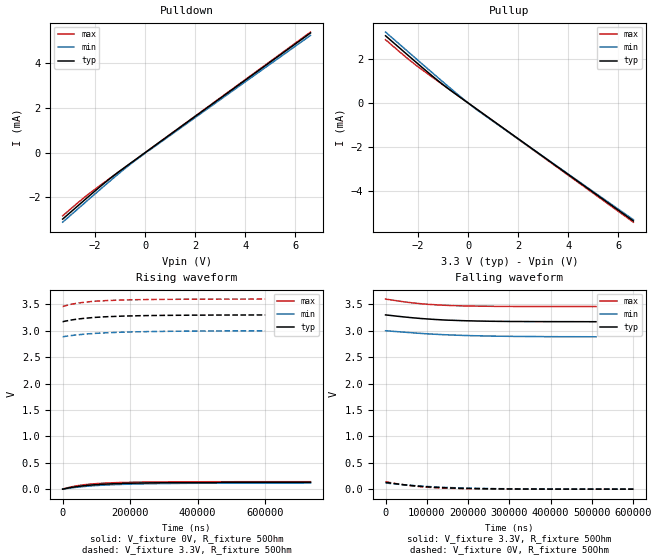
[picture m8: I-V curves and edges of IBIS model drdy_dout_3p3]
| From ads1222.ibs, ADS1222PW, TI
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|   drdy_dout_3p3 Model
[Model]   drdy_dout_3p3
Model_type   Output
Polarity   Non-Inverting
Vmeas = 1.65
Vref = 1.65
Cref = 2pF
Rref = 50
|   typ   min   max
|   (nom PVT)   (fast PVT)   (slow PVT)
|C_comp from frequency sweep method (F= 2.5MHz)
|Average
|C_comp   7.50e-15   6.37e-15   9.00e-15
|ON state : BUFFER OUTPUT TURNED HIGH
C_comp   5.929e-15   5.016e-15   7.087e-15
|OFF state: BUFFER IN HIGH IMPEDANCE
|C_comp   9.065e-15   7.724e-15   1.091e-14
|C_comp from LC tank measurement(L=1nH)
|Average
|Resonant Frequency(Hz)   1.000e+12   1.000e+12   1.000e+12
|C_comp   2.536e-17   2.536e-17   2.536e-17
|ON state : BUFFER OUTPUT TURNED HIGH
|Resonant Frequency(Hz)   1.000e+12   1.000e+12   1.000e+12
|C_comp   2.536e-17   2.536e-17   2.536e-17
|OFF state: BUFFER IN HIGH IMPEDANCE
|Resonant Frequency(Hz)   1.000e+12   1.000e+12   1.000e+12
|C_comp   2.536e-17   2.536e-17   2.536e-17
| Where nom  PVT is Nominal Process, 3.3V, 25C
|   Fast PVT is Strong Process,  3.6V, -40C
|   Slow PVT is Weak Process,   3V, 85C
[Voltage Range]   3.3   3   3.6
|Ambient Temperature   25   85   -40
|Junction Temperature
[Temperature Range]   25   85   -40
[Pullup Reference]   3.3   3   3.6
[Pulldown Reference]   0   0   0
[Power Clamp Reference]   3.3   3   3.6
[GND Clamp Reference]   0   0   0
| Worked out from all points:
|   slope of the pulldown table from 0 to 0.495 V, typ, clamps not added: 1.22 kohm
|   slope of the pullup table from 0 to 0.495 V, typ, clamps not added: 1.23 kohm
|   falling waveform, V_fixture 3.3V, R_fixture 50Ohm: 20-80 % time 137us typ, 162us min, 108us max; typ from 3.3 V to 3.17 V
|   rising waveform, V_fixture 0V, R_fixture 50Ohm: 20-80 % time 131us typ, 165us min, 105us max; typ from 0 V to 0.128 V
|   rising waveform, V_fixture 3.3V, R_fixture 50Ohm: 20-80 % time 144us typ, 172us min, 116us max; typ from 3.17 V to 3.3 V
|   falling waveform, V_fixture 0V, R_fixture 50Ohm: 20-80 % time 122us typ, 152us min, 99.9us max; typ from 0.128 V to 0 V
[Pulldown]
|   Voltage   I(typ)   I(min)   I(max)
-3.3V     -2.986mA   -3.125mA   -2.84mA
-2.281V   -1.988mA   -2.124mA   -1.876mA
-1.468V   -1.218mA   -1.335mA   -1.201mA
-735mV    -596.5uA   -647.6uA   -600uA
-3mV      -401.7nA   -31.96uA   -114.9nA
0V        0A         0A         0A
171mV     141.2uA    108uA      142.7uA
6.6V      5.369mA    5.26mA     5.409mA
[Pullup]
|   Voltage   I(typ)   I(min)   I(max)
-3.3V     3.04mA     3.207mA    2.861mA
-2.166V   1.926mA    2.087mA    1.78mA
-1.178V   982.5uA    1.118mA    961.1uA
309mV     -252.6uA   -280.8uA   -255.6uA
6.6V      -5.341mA   -5.284mA   -5.398mA
[Ramp]
R_load = 50
|   typ   min   max
dV/dt_r   0.0769868/0.00013148   0.0689961/0.000167081  0.0848107/0.000105463
dV/dt_f   0.0773771/0.000134727  0.0685263/0.000168961  0.0849902/0.000107492
[Falling Waveform]
V_fixture = 3.3V
V_fixture_min = 3V
V_fixture_max = 3.6V
R_fixture = 50Ohm
|  time   V(typ)   V(min)   V(max)
0s        3.3V       3V         3.6V
43.71us   3.262V     2.974V     3.549V
64.78us   3.246V     2.962V     3.528V
85.1us    3.232V     2.95V      3.512V
103.6us   3.222V     2.941V     3.5V
132.9us   3.208V     2.929V     3.486V
162.1us   3.198V     2.919V     3.476V
221.9us   3.184V     2.905V     3.466V
311.8us   3.175V     2.893V     3.46V
510.1us   3.171V     2.886V     3.458V
[Rising Waveform]
V_fixture = 0V
V_fixture_min = 0V
V_fixture_max = 0V
R_fixture = 50Ohm
|  time   V(typ)   V(min)   V(max)
0s        24.44uV    0V         24.77uV
13.66us   18.36mV    13.3mV     25.43mV
27.25us   33.81mV    24.99mV    46.12mV
45.69us   51.89mV    39.03mV    67.91mV
64.78us   66.33mV    50.93mV    84.64mV
107.5us   88.53mV    71.42mV    108.5mV
162.1us   105mV      87.61mV    124.2mV
260.2us   119mV      103.3mV    135.5mV
369.3us   124.8mV    110.8mV    139.6mV
735us     128.2mV    116.7mV    141.3mV
[Rising Waveform]
V_fixture = 3.3V
V_fixture_min = 3V
V_fixture_max = 3.6V
R_fixture = 50Ohm
|  time   V(typ)   V(min)   V(max)
0s        3.171V     2.886V     3.458V
13.66us   3.189V     2.899V     3.484V
27.25us   3.205V     2.91V      3.504V
64.78us   3.236V     2.935V     3.54V
107.5us   3.257V     2.954V     3.564V
148.8us   3.27V      2.966V     3.576V
221.9us   3.284V     2.98V      3.588V
311.8us   3.292V     2.989V     3.595V
434.6us   3.297V     2.996V     3.598V
600.6us   3.299V     2.999V     3.6V
[Falling Waveform]
V_fixture = 0V
V_fixture_min = 0V
V_fixture_max = 0V
R_fixture = 50Ohm
|  time   V(typ)   V(min)   V(max)
0s        128.3mV    116.7mV    141.4mV
27.25us   99.94mV    95.72mV    103mV
45.69us   82.58mV    82.6mV     80.88mV
64.78us   67.14mV    70.39mV    62.09mV
85.1us    53.58mV    58.9mV     46.37mV
107.5us   41.39mV    47.73mV    33.35mV
162.1us   21.74mV    28.53mV    14.76mV
221.9us   10.36mV    15.84mV    6.199mV
311.8us   3.508mV    6.269mV    1.615mV
600.6us   118.7uV    12.76uV    43.8uV
